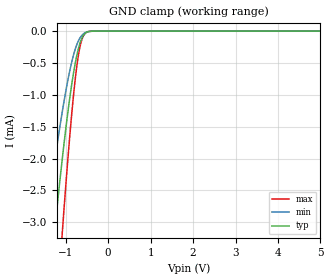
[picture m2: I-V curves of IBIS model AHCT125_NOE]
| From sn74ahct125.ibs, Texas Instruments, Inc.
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[Model]   AHCT125_NOE
Model_type  Input
Vinl=0.8
Vinh=2.0
| variable   typ   min   max
C_comp   0.97pF   0.84pF   1.05pF
[Temperature Range]   40   100   -40
| Ambient temperature   25   85   -40
[Voltage range]   5   4.5   5.5
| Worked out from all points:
|   GND clamp passes 1 mA (typ) near -0.89 V on its own axis
[GND Clamp]
| AHCT125_NOE
|   Voltage   I(typ)   I(min)   I(max)
-5V       -39.32mA   -26.95mA   -49.03mA
-1.49V    -4.776mA   -3.167mA   -7.252mA
-1.26V    -3.141mA   -2.046mA   -4.886mA
-1.085V   -2.032mA   -1.284mA   -3.204mA
-1.06V    -1.885mA   -1.184mA   -2.976mA
-885mV    -959.1uA   -564.7uA   -1.501mA
-760mV    -452.2uA   -252.8uA   -666.7uA
-705mV    -286.8uA   -160.1uA   -398uA
-645mV    -153.5uA   -89.21uA   -193.6uA
-595mV    -80.48uA   -50.51uA   -91.48uA
-520mV    -24.85uA   -17.67uA   -23.13uA
5V        17.64nA    1.142nA    163.4nA
